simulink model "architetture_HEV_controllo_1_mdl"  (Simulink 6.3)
settings: Solver=ode45  StartTime=0.0  StopTime=8  RelTol=1e-3
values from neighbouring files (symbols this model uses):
  b_c = kb*J_c    (= 4.94590955184)    [architetture_epicicloidale.m]    (also in architetture_epicicloidale_cont.m; architetture_epicicloidale_HEV.m = 92.8974810391; architetture_epicicloidale_prova.m; architetture_HEV_controllo.m = 9.28974810391)
  b_p = kb*J_p    (= 8.12277148259)    [architetture_epicicloidale_HEV.m]    (also in architetture_HEV_controllo.m = 0.812277148259; architetture_HEV_startstop.m = 0.0731049433433; Confronto_CVT_EMR.m = 0; epicicloidale_confronto_statico_elastico.m)
  b_r = kb*J_r    (= 218.026030555)    [architetture_epicicloidale.m]    (also in architetture_epicicloidale_cont.m; architetture_epicicloidale_HEV.m; architetture_epicicloidale_prova.m; architetture_HEV_controllo.m = 21.8026030555)
  b_s = kb*J_s    (= 8.12277148259)    [architetture_epicicloidale.m]    (also in architetture_epicicloidale_cont.m; architetture_epicicloidale_HEV.m = 4.94590955184; architetture_epicicloidale_prova.m; architetture_HEV_controllo.m = 0.494590955184)
  bm = 0.8*N*metri*secondo/rad    (= 0.8)    [architetture_epicicloidale.m]    (also in architetture_epicicloidale_cont.m; architetture_epicicloidale_HEV.m; architetture_epicicloidale_prova.m; architetture_HEV_controllo.m)
  d_cr = d0    (= 10)    [architetture_epicicloidale_HEV.m]    (also in architetture_HEV_controllo.m = 1000; architetture_HEV_startstop.m = 90; epicicloidale_confronto_statico_elastico.m; epicicloidale_statico.m)
  d_sc = d0    (= 10)    [architetture_epicicloidale_HEV.m]    (also in architetture_HEV_controllo.m = 1000; architetture_HEV_startstop.m = 90; epicicloidale_confronto_statico_elastico.m; epicicloidale_statico.m)
  I_m = eye(m-1)    [architetture_epicicloidale.m]    (also in architetture_epicicloidale_cont.m; architetture_epicicloidale_HEV.m; architetture_epicicloidale_prova.m; architetture_HEV_controllo.m)
  Iw0 = 0*wI0    [architetture_epicicloidale.m]    (also in architetture_epicicloidale_cont.m = wI0; architetture_epicicloidale_HEV.m; architetture_epicicloidale_prova.m; architetture_HEV_controllo.m)
  J_c = 1.3*0.5*pi*rho_acc*hc*r_c^4    (= 0.0494590955184)    [architetture_epicicloidale.m]    (also in architetture_epicicloidale_cont.m; architetture_epicicloidale_HEV.m = 0.928974810391; architetture_epicicloidale_prova.m; architetture_HEV_controllo.m = 0.928974810391)
  J_p = Nr_sat*0.5*pi*rho_acc*(hs*r_p^4 + hc*r_p^4)    (= 0.0812277148259)    [architetture_epicicloidale_HEV.m]    (also in architetture_HEV_controllo.m; architetture_HEV_startstop.m; Confronto_CVT_EMR.m = 0; epicicloidale_confronto_statico_elastico.m)
  J_r = 0.5*pi*rho_acc*(hr*r_ri^4 + h_ring*(r_re^4-r_ri^4))    (= 2.18026030555)    [architetture_epicicloidale.m]    (also in architetture_epicicloidale_cont.m; architetture_epicicloidale_HEV.m; architetture_epicicloidale_prova.m; architetture_HEV_controllo.m)
  J_s = Nr_sat*0.5*pi*rho_acc*(hs*r_s^4 + hc*r_s^4)    (= 0.0812277148259)    [architetture_epicicloidale.m]    (also in architetture_epicicloidale_cont.m; architetture_epicicloidale_HEV.m = 0.0494590955184; architetture_epicicloidale_prova.m; architetture_HEV_controllo.m = 0.0494590955184)
  Jm = 1.6*kg*metri^2    (= 1.6)    [architetture_epicicloidale.m]    (also in architetture_epicicloidale_cont.m; architetture_epicicloidale_HEV.m = 1.64945909552; architetture_epicicloidale_prova.m; architetture_HEV_controllo.m = 0.529459095518)
  Jr = Jr([1:m-1],[1:m-1])    [architetture_epicicloidale.m]    (also in architetture_epicicloidale_cont.m; architetture_epicicloidale_HEV.m; architetture_epicicloidale_prova.m; architetture_HEV_controllo.m)
  K_cr = K0    (= 10000)    [architetture_epicicloidale_HEV.m]    (also in architetture_HEV_controllo.m = 100000; architetture_HEV_startstop.m = 10000000; epicicloidale_confronto_statico_elastico.m; epicicloidale_statico.m)
  K_sc = K0    (= 10000)    [architetture_epicicloidale_HEV.m]    (also in architetture_HEV_controllo.m = 100000; architetture_HEV_startstop.m = 10000000; epicicloidale_confronto_statico_elastico.m; epicicloidale_statico.m)
  Kf = diag(diag(MLb)'./fliplr(tau_m(1:m-1)))    [architetture_epicicloidale_cont.m]    (also in architetture_epicicloidale_HEV.m; architetture_epicicloidale_prova.m; architetture_HEV_controllo.m; architetture_HEV_startstop.m)
  km = 1000*metri    (= 1000)    [architetture_epicicloidale.m]    (also in architetture_epicicloidale_cont.m; architetture_epicicloidale_HEV.m; architetture_epicicloidale_prova.m; architetture_HEV_controllo.m)
  Kprop = 32.3*5    (= 161.5)    [architetture_HEV_controllo.m]    (also in architetture_HEV_startstop.m; PMSM_controllo_w.m = 32.3; architetture_HEV_startstop_1.m; architetture_HEV_startstop_2.m)
  Kr = Kr([1:m-1])    [architetture_epicicloidale.m]    (also in architetture_epicicloidale_cont.m; architetture_epicicloidale_HEV.m; architetture_epicicloidale_prova.m; architetture_HEV_controllo.m)
  Li = 0.1*Henry    (= 0.1)    [architetture_epicicloidale.m]    (also in architetture_epicicloidale_cont.m; architetture_epicicloidale_HEV.m; architetture_epicicloidale_prova.m; architetture_HEV_controllo.m)
  m = 5    [architetture_epicicloidale.m]    (also in architetture_epicicloidale_cont.m; architetture_epicicloidale_HEV.m; architetture_epicicloidale_prova.m; architetture_HEV_controllo.m)
  Mi = 0.08*Henry    (= 0.08)    [architetture_epicicloidale.m]    (also in architetture_epicicloidale_cont.m; architetture_epicicloidale_HEV.m; architetture_epicicloidale_prova.m; architetture_HEV_controllo.m)
  MKr = MKr([1:m-1],[1:m-1])    [architetture_epicicloidale.m]    (also in architetture_epicicloidale_cont.m; architetture_epicicloidale_HEV.m; architetture_epicicloidale_prova.m; architetture_HEV_controllo.m)
  MLb = MLb([1:m-1],[1:m-1])    [architetture_epicicloidale.m]    (also in architetture_epicicloidale_cont.m; architetture_epicicloidale_HEV.m; architetture_epicicloidale_prova.m; architetture_HEV_controllo.m)
  MR = MR([1:m-1],[1:m-1])    [architetture_epicicloidale.m]    (also in architetture_epicicloidale_cont.m; architetture_epicicloidale_HEV.m; architetture_epicicloidale_prova.m; architetture_HEV_controllo.m)
  Nar = 200    [architetture_epicicloidale.m]    (also in architetture_epicicloidale_cont.m; architetture_epicicloidale_HEV.m; architetture_epicicloidale_prova.m; architetture_HEV_controllo.m)
  Nc = 30    [architetture_epicicloidale.m]    (also in architetture_epicicloidale_cont.m; architetture_epicicloidale_HEV.m; architetture_epicicloidale_prova.m; architetture_HEV_controllo.m)
  Nr_sat = 4    [architetture_epicicloidale.m]    (also in architetture_epicicloidale_cont.m; architetture_epicicloidale_HEV.m; architetture_epicicloidale_prova.m; architetture_HEV_controllo.m)
  ora = 60*60*secondo    (= 3600)    [architetture_epicicloidale.m]    (also in architetture_epicicloidale_cont.m; architetture_epicicloidale_HEV.m; architetture_epicicloidale_prova.m; architetture_HEV_controllo.m)
  p = 1    [architetture_epicicloidale.m]    (also in architetture_epicicloidale_cont.m; architetture_epicicloidale_HEV.m; architetture_epicicloidale_prova.m; architetture_HEV_controllo.m)
  Phir = 0.02*Weber    (= 0.02)    [architetture_epicicloidale.m]    (also in architetture_epicicloidale_cont.m; architetture_epicicloidale_HEV.m; architetture_epicicloidale_prova.m; architetture_HEV_controllo.m)
  r_p = xds*Np/(2*pi)    (= 0.0732112738223)    [architetture_epicicloidale_HEV.m]    (also in architetture_HEV_controllo.m; architetture_HEV_startstop.m; Confronto_CVT_EMR.m = 0.025; epicicloidale_confronto_statico_elastico.m)
  r_r = xds*Nr/(2*pi)    (= 0.248281711223)    [architetture_epicicloidale_HEV.m]    (also in architetture_HEV_controllo.m; architetture_HEV_startstop.m; Confronto_CVT_EMR.m = 0.1; epicicloidale_confronto_statico_elastico.m)
  r_s = xds*Ns/(2*pi)    (= 0.0732112738223)    [architetture_epicicloidale.m]    (also in architetture_epicicloidale_cont.m; architetture_epicicloidale_HEV.m = 0.101859163579; architetture_epicicloidale_prova.m; architetture_HEV_controllo.m = 0.101859163579)
  Ri = 3*Ohm    (= 3)    [architetture_epicicloidale.m]    (also in architetture_epicicloidale_cont.m; architetture_epicicloidale_HEV.m; architetture_epicicloidale_prova.m; architetture_HEV_controllo.m = 0.1)
  Star = Si    [architetture_epicicloidale.m]    (also in architetture_epicicloidale_cont.m; architetture_epicicloidale_HEV.m; architetture_epicicloidale_prova.m; architetture_HEV_controllo.m)
  Tc = 0.05*ms    (= 5e-05)    [architetture_epicicloidale.m]    (also in architetture_epicicloidale_cont.m; architetture_epicicloidale_HEV.m; architetture_epicicloidale_prova.m; architetture_HEV_controllo.m)
  Tc_0 = 0*N*metri    (= 0)    [architetture_epicicloidale_HEV.m]    (also in architetture_HEV_controllo.m; architetture_HEV_startstop.m; epicicloidale_confronto_statico_elastico.m; epicicloidale_statico.m)
  Tder = 0.0119*20    (= 0.238)    [architetture_HEV_controllo.m]    (also in architetture_HEV_startstop.m; PMSM_controllo_w.m; architetture_HEV_startstop_1.m; architetture_HEV_startstop_2.m)
  Thm0 = 0    [architetture_epicicloidale.m]    (also in architetture_epicicloidale_cont.m; architetture_epicicloidale_HEV.m; architetture_epicicloidale_prova.m; architetture_HEV_controllo.m)
  Tint = 0.2427*10    (= 2.427)    [architetture_HEV_controllo.m]    (also in architetture_HEV_startstop.m; PMSM_controllo_w.m = 0.2427; architetture_HEV_startstop_1.m; architetture_HEV_startstop_2.m)
  Tr_0 = 0*N*metri    (= 0)    [architetture_epicicloidale_HEV.m]    (also in architetture_HEV_controllo.m; architetture_HEV_startstop.m; epicicloidale_confronto_statico_elastico.m; epicicloidale_statico.m)
  Ts = Tfin/2000    (= 0.00025)    [architetture_epicicloidale.m]    (also in architetture_epicicloidale_cont.m = 0.001; architetture_epicicloidale_HEV.m = 0.0025; architetture_epicicloidale_prova.m = 0.001; architetture_HEV_controllo.m = 0.004)
  Ts_0 = 0*N*metri    (= 0)    [architetture_epicicloidale_HEV.m]    (also in architetture_HEV_controllo.m; architetture_HEV_startstop.m; epicicloidale_confronto_statico_elastico.m; epicicloidale_statico.m)
  tTb = tTb(:,[1:m-1])    [architetture_epicicloidale.m]    (also in architetture_epicicloidale_cont.m; architetture_epicicloidale_HEV.m; architetture_epicicloidale_prova.m; architetture_HEV_controllo.m)
  Wc_0 = 0*0.1*rad/secondo    (= 0)    [architetture_epicicloidale.m]    (also in architetture_epicicloidale_cont.m; architetture_epicicloidale_HEV.m; architetture_epicicloidale_prova.m; Confronto_CVT_EMR.m)
  Wm0 = 0*Wr_d    (= 0)    [architetture_epicicloidale.m]    (also in architetture_epicicloidale_cont.m = 62.5; architetture_epicicloidale_HEV.m; architetture_epicicloidale_prova.m; architetture_HEV_controllo.m)
  Wr_0 = Sys1.C(3,:)*[Wc_0; Wsc_0]    [architetture_epicicloidale.m]    (also in Confronto_CVT_EMR.m = 0; epicicloidale.m; epicicloidale_confronto_statico_elastico.m = [-r_s/r_r, 1+r_s/r_r]*[Ws_0; Wc_0]; epicicloidale_da_solo.m = [ -1/r_ri*r_c, (r_c+r_ri)/r_ri]*[Wc_0; Wsc_0])
  Ws_0 = 0.1*rad/secondo    (= 0.1)    [epicicloidale_confronto_statico_elastico.m]    (also in epicicloidale_statico.m; architetture_epicicloidale_statico.m = 0)
undefined symbols (not defined in the file or in its folder): Wc, Wr
libraries: simulink x2, planetary_gear_blocks x2, POG_Sincronous_Motors x1

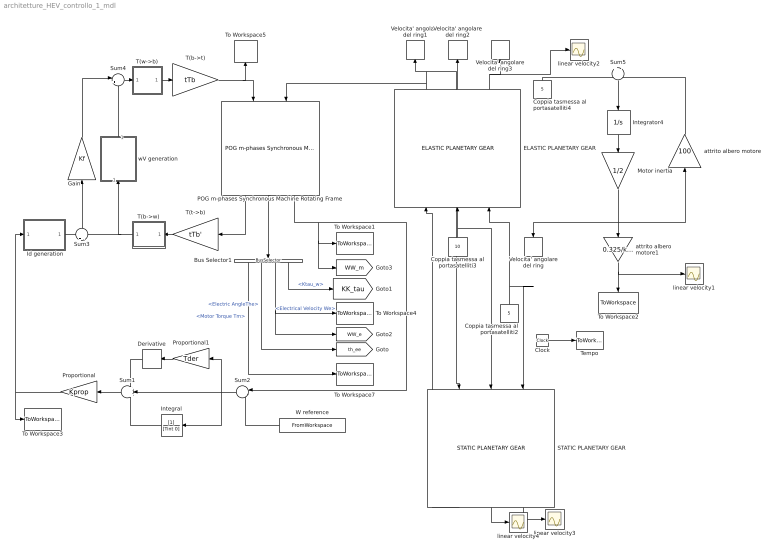
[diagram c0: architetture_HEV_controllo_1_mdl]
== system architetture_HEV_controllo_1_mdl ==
  " Id generation" : Subsystem
  Bus Selector1 : BusSelector  Orientation=down  OutputSignals=Motor Torque Tm,Electric AngleThe,Electrical Velocity We,Ktau_w
  Clock : Clock
  Coppia tasmessa al portasatelliti2 : Constant  Orientation=up  Value=5
  Coppia tasmessa al portasatelliti3 : Constant  Orientation=up  Value=10
  Coppia tasmessa al portasatelliti4 : Constant  Orientation=up  Value=5
  Derivative : Derivative  Orientation=left
  ELASTIC PLANETARY GEAR : planetary_gear_blocks/ELASTIC PLANETARY GEAR  Orientation=up  Par_solare=[J_s, b_s, r_s]  Par_satelliti=[J_p, J_c, b_p, b_c, r_p, Nr_sat]  Par_ring=[J_r, b_r, r_r]  Solare_Satelliti=[K_sc, d_sc]  Satelliti_Ring=[K_cr, d_cr]  Cond_in=[Ts_0, Tc_0, Tr_0]
  Gain : Gain  Orientation=up  Gain=Kf  Multiplication=Matrix(K*u) (u vector)
  Integral : TransferFcn  Orientation=left  Denominator=[Tint 0]
  Integrator4 : Integrator  Orientation=down  InitialCondition=Wm0*Jm
  Motor inertia : Gain  Orientation=down  Gain=1/2
  POG m-phases Synchronous Machine Rotating Frame : POG_Sincronous_Motors/POG m-phases Synchronous Machine Rotating Frame  Orientation=down  Motor_Par=[m p]  Phase_Par=[Nc Star]  Electric_Par=[Ri Li Mi]  Mech_Par=[Jm bm]  Plux_Par=[Phir Nar]  Iniz_Cond=[Wm0; Thm0; Iw0]  TipoFlux=User defined  Tipo=Tipo  alfa=al  degree=6  TipoF=Tipo
  Proportional : Gain  Orientation=left  Gain=Kprop
  Proportional1 : Gain  Orientation=left  Gain=Tder
  STATIC PLANETARY GEAR : planetary_gear_blocks/STATIC PLANETARY GEAR  Orientation=down  Raggi_sun_ring=[r_s, r_r]  Tipo_di_Modello=Ts-Wc-Wr  Cond_in_Ws_Wc="[Ws_0,  Wc_0]"  Cond_in_Wc_Wr="[0,  0]"  Cond_in_Ws_Wr="[Ws_0,  Wr_0]"  Cond_in=[Ws_0, Wc_0, Wr_0]
  Sum1 : Sum  Orientation=left  Inputs=+++
  Sum2 : Sum  Orientation=left  Inputs=|-+
  Sum3 : Sum  Orientation=up  Inputs=+|-
  Sum4 : Sum  Inputs=|++
  Sum5 : Sum  Orientation=down  Inputs=+|-
  T(b->t) : Gain  Gain=tTb  Multiplication=Matrix(K*u) (u vector)
  T(b->w) : Subsystem  Orientation=left  AncestorBlock=|
      | POG_Electric_Bloks/POG m-phases
      | Synchronous Machine
      | Rotating Frame/T(b->w)
  T(t->b) : Gain  Orientation=left  Gain=tTb'  Multiplication=Matrix(K*u) (u vector)
  T(w->b) : Subsystem  AncestorBlock=|
      | POG_Electric_Bloks/POG m-phases
      | Synchronous Machine
      | Rotating Frame/T(w->b)
  Tempo : ToWorkspace  VariableName=t  SampleTime=Tc  SaveFormat=Array
  To Workspace1 : ToWorkspace  VariableName=Wm  SampleTime=Tc  SaveFormat=Array
  To Workspace2 : ToWorkspace  VariableName=Vvehicle  SampleTime=Tc  SaveFormat=Array
  To Workspace3 : ToWorkspace  VariableName=Tref  SampleTime=Tc  SaveFormat=Array
  To Workspace4 : ToWorkspace  VariableName=We  SampleTime=Tc  SaveFormat=Array
  To Workspace5 : ToWorkspace  VariableName=Vt  SampleTime=Tc  SaveFormat=Array
  To Workspace7 : ToWorkspace  VariableName=Tm  SampleTime=Tc  SaveFormat=Array
  Velocita' angolare del ring : ToWorkspace  VariableName=W_r  SampleTime=Tc  SaveFormat=Array
  Velocita' angolare del ring1 : ToWorkspace  VariableName=Tau_s  SampleTime=Tc  SaveFormat=Array
  Velocita' angolare del ring2 : ToWorkspace  VariableName=Tau_c  SampleTime=Tc  SaveFormat=Array
  Velocita' angolare del ring3 : ToWorkspace  VariableName=Tau_r  SampleTime=Tc  SaveFormat=Array
  W reference : FromWorkspace  Orientation=left  VariableName=[T_in W_sun_des]  SampleTime=0
  attrito albero motore : Gain  Orientation=up  Gain=100
  attrito albero motore1 : Gain  Orientation=down  Gain=0.325/km*ora
  linear velocity{1..4} (4 alike) : Scope
  wV generation : Subsystem  Orientation=up
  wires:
  Clock/1 -> Tempo/1
  POG m-phases Synchronous Machine Rotating Frame/3 -> To Workspace1/1, [WW_m], Sum2/1
  POG m-phases Synchronous Machine Rotating Frame/2 -> Bus Selector1/1
  Bus Selector1/3 -> To Workspace4/1, [WW_e]  "<Electrical Velocity We>"
  T(w->b)/1(It) -> T(b->t)/1
  T(b->t)/1 -> POG m-phases Synchronous Machine Rotating Frame/1, To Workspace5/1
  T(t->b)/1 -> T(b->w)/1(Vt)
  T(b->w)/1(Vw) -> wV generation/1(In1), Sum3/2
  POG m-phases Synchronous Machine Rotating Frame/1 -> T(t->b)/1
  Bus Selector1/2 -> [th_ee]  "<Electric AngleThe>"
  Bus Selector1/1 -> To Workspace7/1  "<Motor Torque Tm>"
  " Id generation"/1(Out1) -> Sum3/1
  Sum3/1 -> Gain/1
  Sum4/1 -> T(w->b)/1(Iw)
  Gain/1 -> Sum4/1
  wV generation/1(Out1) -> Sum4/2
  Bus Selector1/4 -> [KK_tau]  "<Ktau_w>"
  ELASTIC PLANETARY GEAR/3 -> Velocita' angolare del ring3/1, linear velocity2/1
  ELASTIC PLANETARY GEAR/1 -> POG m-phases Synchronous Machine Rotating Frame/2, Velocita' angolare del ring1/1, STATIC PLANETARY GEAR/1
  ELASTIC PLANETARY GEAR/2 -> Velocita' angolare del ring2/1
  Coppia tasmessa al portasatelliti3/1 -> ELASTIC PLANETARY GEAR/2, STATIC PLANETARY GEAR/2
  Sum2/1 -> Integral/1, Proportional1/1, Sum1/2
  W reference/1 -> Sum2/2
  Sum1/1 -> Proportional/1
  Proportional1/1 -> Derivative/1
  Derivative/1 -> Sum1/1
  Integral/1 -> Sum1/3
  Proportional/1 -> " Id generation"/1(In1), To Workspace3/1
  Integrator4/1 -> Motor inertia/1
  Sum5/1 -> Integrator4/1
  attrito albero motore/1 -> Sum5/2
  Motor inertia/1 -> attrito albero motore/1, attrito albero motore1/1, Velocita' angolare del ring/1
  attrito albero motore1/1 -> To Workspace2/1, linear velocity1/1
  Coppia tasmessa al portasatelliti4/1 -> Sum5/1
  Coppia tasmessa al portasatelliti2/1 -> ELASTIC PLANETARY GEAR/3, STATIC PLANETARY GEAR/3
  STATIC PLANETARY GEAR/1 -> ELASTIC PLANETARY GEAR/1
  STATIC PLANETARY GEAR/3 -> linear velocity3/1
  STATIC PLANETARY GEAR/2 -> linear velocity4/1

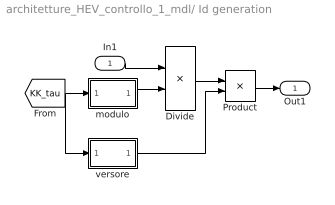
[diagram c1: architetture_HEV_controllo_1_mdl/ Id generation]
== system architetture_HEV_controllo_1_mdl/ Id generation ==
  In1 : Inport
  Divide : Product  Inputs=*/  OutScaling=2^-10
  Product : Product
  modulo : Subsystem
  versore : Subsystem
  Out1 : Outport
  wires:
  [KK_tau] -> modulo/1(In1), versore/1(In1)
  modulo/1(Out1) -> Divide/2
  Divide/1 -> Product/1
  versore/1(Out1) -> Product/2
  In1/1 -> Divide/1
  Product/1 -> Out1/1

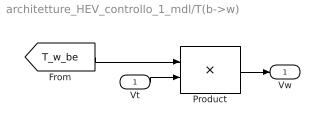
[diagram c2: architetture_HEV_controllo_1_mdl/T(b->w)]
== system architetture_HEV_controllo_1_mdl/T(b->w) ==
  Vt : Inport
  Product : Product  Multiplication=Matrix(*)
  Vw : Outport
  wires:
  Vt/1 -> Product/2
  Product/1 -> Vw/1
  [T_w_be] -> Product/1

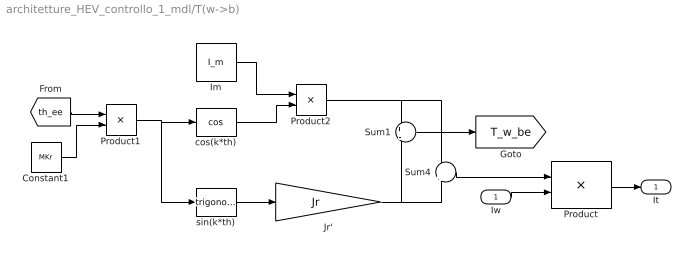
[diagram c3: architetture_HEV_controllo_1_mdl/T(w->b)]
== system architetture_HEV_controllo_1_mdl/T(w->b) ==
  Iw : Inport
  Constant1 : Constant  Value=MKr
  Im : Constant  Value=I_m  VectorParams1D=off
  Jr' : Gain  Gain=Jr  Multiplication=Matrix(K*u)
  Product : Product  Multiplication=Matrix(*)
  Product1 : Product
  Product2 : Product
  Sum1 : Sum  Inputs=+|-
  Sum4 : Sum  Inputs=+|+
  cos(k*th) : Trigonometry  Operator=cos
  sin(k*th) : Trigonometry
  It : Outport
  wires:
  Sum4/1 -> Product/1
  Product/1 -> It/1
  Iw/1 -> Product/2
  Jr'/1 -> Sum4/2, Sum1/2
  Product2/1 -> Sum4/1, Sum1/1
  Im/1 -> Product2/1
  cos(k*th)/1 -> Product2/2
  Product1/1 -> sin(k*th)/1, cos(k*th)/1
  Constant1/1 -> Product1/2
  [th_ee] -> Product1/1
  sin(k*th)/1 -> Jr'/1
  Sum1/1 -> [T_w_be]

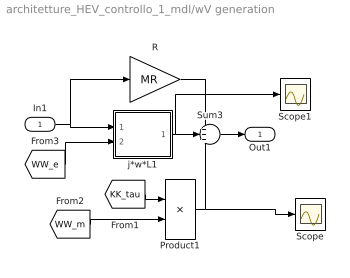
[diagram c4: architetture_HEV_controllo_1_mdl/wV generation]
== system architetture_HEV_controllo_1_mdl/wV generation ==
  In1 : Inport
  Product1 : Product  Multiplication=Matrix(*)
  R : Gain  Gain=MR  Multiplication=Matrix(K*u) (u vector)
  Scope : Scope
  Scope1 : Scope
  Sum3 : Sum  Inputs=+++
  j*w*L1 : Subsystem  AncestorBlock=|
      | POG_Electric_Bloks/POG m-phases
      | Synchronous Machine
      | Rotating Frame/j*w*L
  Out1 : Outport
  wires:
  [KK_tau] -> Product1/1
  [WW_m] -> Product1/2
  R/1 -> Sum3/1
  j*w*L1/1(Out1) -> Sum3/2, Scope1/1
  Product1/1 -> Sum3/3, Scope/1
  In1/1 -> j*w*L1/1(In1), R/1
  Sum3/1 -> Out1/1
  [WW_e] -> j*w*L1/2(In2)

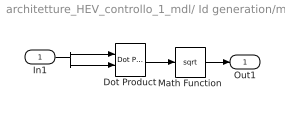
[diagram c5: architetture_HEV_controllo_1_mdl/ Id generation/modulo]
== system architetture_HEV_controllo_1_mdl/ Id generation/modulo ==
  In1 : Inport
  Dot Product : simulink/Math Operations/Dot Product  InputSameDT=on  OutDataType=sfix(16)  OutScaling=2^-10  DoSatur=off
  Math Function : Math  Operator=sqrt
  Out1 : Outport
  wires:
  In1/1 -> Dot Product/1, Dot Product/2
  Dot Product/1 -> Math Function/1
  Math Function/1 -> Out1/1

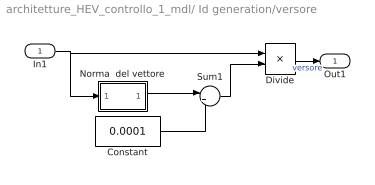
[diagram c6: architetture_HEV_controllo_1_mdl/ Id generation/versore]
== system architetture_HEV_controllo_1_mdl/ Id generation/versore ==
  In1 : Inport
  Constant : Constant  Value=0.0001
  Divide : Product  Inputs=*/  OutScaling=2^-10
  Norma  del vettore : Subsystem
  Sum1 : Sum  Inputs=|++
  Out1 : Outport
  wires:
  Divide/1 -> Out1/1  "versore"
  Constant/1 -> Sum1/2
  Sum1/1 -> Divide/2
  Norma  del vettore/1(Out1) -> Sum1/1
  In1/1 -> Norma  del vettore/1(In1), Divide/1

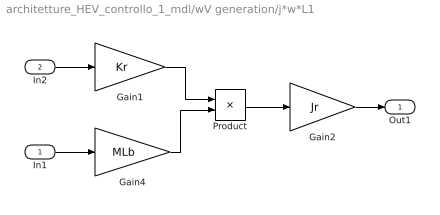
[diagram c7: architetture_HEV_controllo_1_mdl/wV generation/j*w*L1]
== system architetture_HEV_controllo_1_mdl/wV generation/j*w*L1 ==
  In1 : Inport
  In2 : Inport  Port=2
  Gain1 : Gain  Gain=Kr  Multiplication=Matrix(K*u) (u vector)
  Gain2 : Gain  Gain=Jr  Multiplication=Matrix(K*u) (u vector)
  Gain4 : Gain  Gain=MLb  Multiplication=Matrix(K*u) (u vector)
  Product : Product
  Out1 : Outport
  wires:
  In1/1 -> Gain4/1
  In2/1 -> Gain1/1
  Gain1/1 -> Product/1
  Gain4/1 -> Product/2
  Product/1 -> Gain2/1
  Gain2/1 -> Out1/1

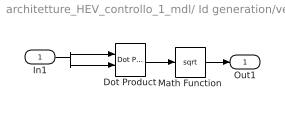
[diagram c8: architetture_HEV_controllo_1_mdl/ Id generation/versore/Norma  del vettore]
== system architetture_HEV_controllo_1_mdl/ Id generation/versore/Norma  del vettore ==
  In1 : Inport
  Dot Product : simulink/Math Operations/Dot Product  InputSameDT=on  OutDataType=sfix(16)  OutScaling=2^-10  DoSatur=off
  Math Function : Math  Operator=sqrt
  Out1 : Outport
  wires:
  Math Function/1 -> Out1/1
  Dot Product/1 -> Math Function/1
  In1/1 -> Dot Product/2, Dot Product/1
